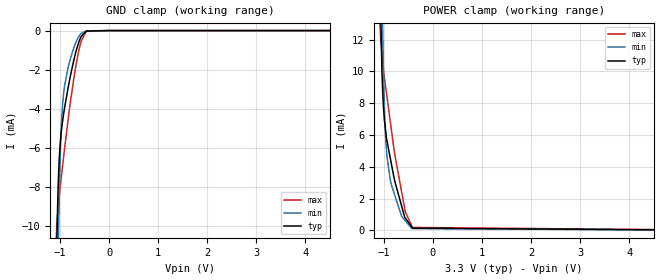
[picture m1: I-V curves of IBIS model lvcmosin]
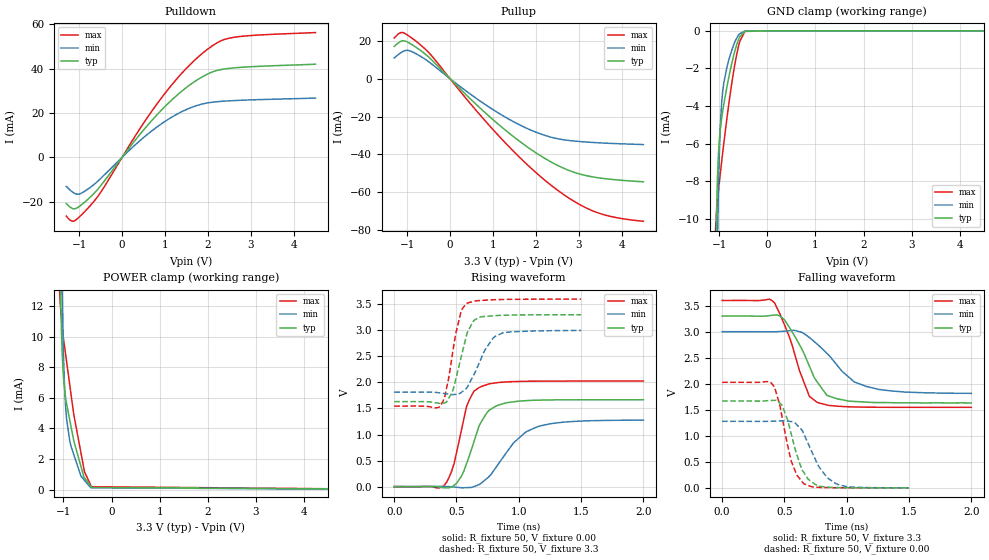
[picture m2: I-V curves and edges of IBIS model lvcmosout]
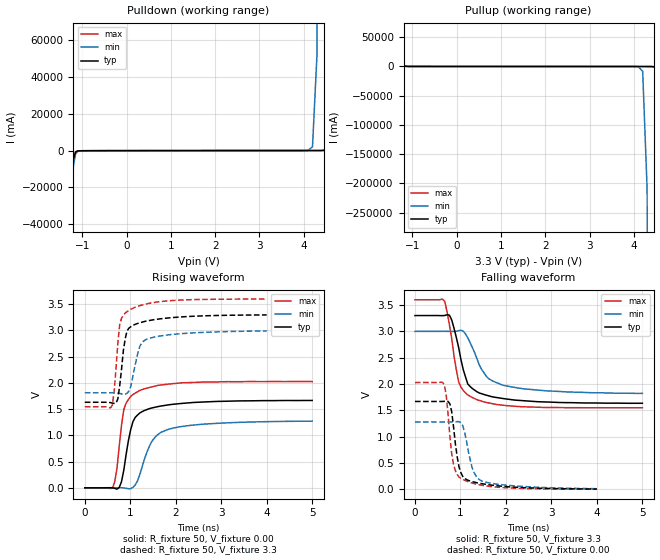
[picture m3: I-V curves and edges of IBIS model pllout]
|Texas Instruments, Incorporated   |
|Four Output Clock Generator/Jitter Cleaner With Integrated Dual VCOs   |
| Marketing part#   Voltage Range   Package-type   #pins/pkg drawing |
| CDCE62002RHBR   3.0V - 3.6V   QFN   32-pin RHB   |
| CDCE62002RHBT   3.0V - 3.6V   QFN   32-pin RHB   |
[IBIS Ver]   4.0
[File name]   cdce62002.ibs
[File Rev]   1.0
[Date]   09/18/2015
[Source]   Texas Instruments Incorporated.
   Analog-eLab, HPA
   12500 TI Blvd
   Dallas, TX -75243
   For Support e-mail: elab_scm_ibis@list.ti.com
[Notes]   Revision History
   Rev 1.0: 09/18/2015
   - Same base die and models as CDCE62005, new package model.
[Disclaimer] This model is designed as an aid for customers of Texas Instruments.
 TI and its licensors and suppliers make no warranties, either expressed
 or implied, with respect to this  model, including the warranties of
 merchantability or fitness for a particular purpose.
 The model is provided solely on an "as is" basis. The entire risk as to
 its quality and performance is with the customer.
[Copyright] (C)Copyright 2015 Texas Instruments Incorporated.
   All rights reserved.
|   Component   CDCE62002RHB
[Component]   CDCE62002RHB
[Manufacturer]   Texas Instruments Incorporated
[Package]   |32-pin RHB Package, QFN
|   typ   min   max
R_pkg   0.1266   0.0917   0.1676
L_pkg   1.089nH   0.7569nH   1.4898nH
C_pkg   0.1201pF   0.0925pF   0.1533pF
[Pin] signal_name   model_name   R_pin   L_pin   C_pin
1   VCC_AUX   POWER   0.00505   0.15571nH   1.25602pF
2   AUX_IN   lvcmosin   0.13153   1.1302nH   0.1258pF
3   VBB   POWER   0.10832   0.90731nH   0.10655pF
4   VCC_PLLD   POWER   0.04958   0.55167nH   0.12597pF
5   REG_CAP1   NC   0.09166   0.75685nH   0.09254pF
6   PDN   lvcmosin   0.09642   0.80223nH   0.09606pF
7   SPI_MISO   lvcmosout   0.11258   0.95481nH   0.10947pF
8   SPI_MOSI   lvcmosin   0.13603   1.18504nH   0.11758pF
9   VCC_OUT0   POWER   0.07038   0.91081nH   0.16021pF
10   U0_N   univoutN   0.13453   1.1681nH   0.12847pF
11   U0_P   univoutP   0.13111   1.13436nH   0.12596pF
12   VCC_OUT1   POWER   0.06752   0.84332nH   0.17642pF
13   VCC_OUT2   POWER   0.06751   0.84583nH   0.17926pF
14   U1_N   univoutN   0.13123   1.13557nH   0.12556pF
15   U1_P   univoutP   0.13419   1.1648nH   0.12877pF
16   VCC_OUT3   POWER   0.0704   0.90108nH   0.16069pF
17   SPI_CLK   lvcmosin   0.13766   1.20093nH   0.1195pF
18   SPI_LE   lvcmosin   0.11212   0.95041nH   0.11038pF
19   TEST_SYNC   NC   0.09475   0.78685nH   0.09573pF
20   REG_CAP3   NC   0.09303   0.76838nH   0.09454pF
21   GND_PLLDIV   GND   0.05226   0.59794nH   0.13463pF
22   VCC_PLLDIV   POWER   0.05772   0.69812nH   0.14663pF
23   REG_CAP4   NC   0.13319   1.1464nH   0.12871pF
24   VCC_VCO   POWER   0.07578   1.10044nH   0.15548pF
25   EXT_LF_P   NC   0.16761   1.48983nH   0.15332pF
26   EXT_LF_N   NC   0.14699   1.2821nH   0.13427pF
27   REG_CAP2   NC   0.13767   1.18956nH   0.13285pF
28   VCC_PLLA   POWER   0.06718   0.82907nH   0.17636pF
29   REF_P   univin   0.13272   1.14077nH   0.12791pF
30   REF_N   univin   0.13255   1.13927nH   0.12699pF
31   VCC_IN   POWER   0.06896   0.86472nH   0.17429pF
32   PLL_LOCK   pllout   0.14347   1.24974nH   0.12652pF
|33   GND_THERMALPAD
[Diff Pin]  inv_pin  vdiff  tdelay_typ tdelay_min tdelay_max
| VDIFF TYP FOR lvds = 410mV; lvpecl_lo = 690mV
|lvpecl_hi = 810mV
11   10   0   NA   NA   NA
15   14   0   NA   NA   NA
29   30   200mV   NA   NA   NA
[Model Selector]   univoutP
univoutc   buffer with LVCMOS
univoutl   buffer with LVDS with normal swing
LVPECL_RC_HI_p LVPECL for HI SWING for positive Pin
LVPECL_RC_LO_p LVPECL for LO SWING for positive pin
[Model Selector]   univoutN
univoutc   buffer with LVCMOS
univoutl   buffer with LVDS with normal swing
LVPECL_RC_HI_n LVPECL for HI SWING for negative Pin
LVPECL_RC_LO_n LVPECL for LO SWING for negative pin
[Model Selector]   univin
univinc   input buffer with LVCMOS with internal termination
univine   input buffer with LVPECL with internal termination
univinl   input buffer with LVDS with internal termination
| Models and submodels in the file (12): lvcmosin (Input), lvcmosout (3-state), pllout (Output), univinc (Input), univinl (Input), univine (Input), univoutc (Output), LVPECL_RC_HI_p (Output_ECL), LVPECL_RC_HI_n (Output_ECL), LVPECL_RC_LO_p (Output_ECL), LVPECL_RC_LO_n (Output_ECL), univoutl (3-state)
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|   Model   lvcmosin
[Model]   lvcmosin
Model_type   Input
Polarity   Non-Inverting
Vinl   =   0.99V
Vinh   =   2.31V
|Variable   typ   min   max
C_comp   6.462e-13   6.387e-13   6.627e-13
[Model Spec]
Vinl   0.99V   0.9V   1.08V
Vinh   2.31V   2.1V   2.52V
|Variable   typ   min   max
[Voltage range]   3.3   3.0   3.6
|Variable   typ   min   max
[Temperature range]  25   85   0
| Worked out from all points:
|   GND clamp passes 1 mA (typ) near -0.67 V on its own axis
|   POWER clamp passes 1 mA (typ) near -0.59 V on its own axis
[GND Clamp]
|   Voltage   I(typ)   I(min)   I(max)
-3.3V     -1.163A    -1.155A    -1.183A
-1.077V   -12.52mA   -19.9mA    -10.51mA
-1.062V   -10.33mA   -16.3mA    -9.851mA
-1.04V    -8.005mA   -11.81mA   -9.112mA
-1.03V    -7.282mA   -10.19mA   -8.835mA
-1.001V   -5.883mA   -6.686mA   -8.1mA
-975.8mV  -5.179mA   -4.92mA    -7.525mA
-948.5mV  -4.618mA   -3.762mA   -6.913mA
-906.5mV  -3.923mA   -2.782mA   -5.998mA
-666.2mV  -976.2uA   -532.3uA   -1.635mA
-473.3mV  -43.09uA   -22.62uA   -64.41uA
6.598V    0A         0A         0A
[POWER Clamp]
|   Voltage   I(typ)   I(min)   I(max)
-3.3V     1.174A     1.165A     1.197A
-1.079V   16.53mA    24.99mA    12.95mA
-1.065V   13.88mA    21.26mA    12.05mA
-1.025V   8.881mA    12.83mA    10.64mA
-1.005V   7.625mA    9.46mA     9.995mA
-990.5mV  6.997mA    7.918mA    9.669mA
-956.5mV  6.058mA    5.501mA    8.88mA
-866.6mV  4.514mA    3.149mA    6.797mA
-778.6mV  3.136mA    2.225mA    4.803mA
-562.5mV  777.7uA    608.5uA    1.165mA
-432.4mV  233.3uA    121.2uA    290.1uA
6.59V     0A         0A         0A
|   Model   lvcmosout
[Model]   lvcmosout
Model_type   3-state
Polarity   Non-Inverting
Enable   Active-Low
Vmeas  =   1.55V
Cref   =   5pF
Vref   =   0V
|Variable   typ   min   max
C_comp   1.519e-12   1.481e-12   1.560e-12
[Model Spec]
Vmeas   1.55V   1.4V   1.7V
|Variable   typ   min   max
[Voltage range]   3.3   3.0   3.6
|Variable   typ   min   max
[Temperature range]  25   85   0
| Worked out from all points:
|   slope of the pulldown table from 0 to 0.495 V, typ, clamps not added: 40.6 ohm
|   slope of the pullup table from 0 to 0.495 V, typ, clamps not added: 44.4 ohm
|   GND clamp passes 1 mA (typ) near -0.67 V on its own axis
|   POWER clamp passes 1 mA (typ) near -0.59 V on its own axis
|   rising waveform, R_fixture 50, V_fixture 0.00: 20-80 % time 158ps typ, 259ps min, 120ps max; typ from 0 V to 1.67 V
|   falling waveform, R_fixture 50, V_fixture 3.3: 20-80 % time 215ps typ, 291ps min, 178ps max; typ from 3.3 V to 1.63 V
|   rising waveform, R_fixture 50, V_fixture 3.3: 20-80 % time 104ps typ, 150ps min, 92.8ps max; typ from 1.63 V to 3.3 V
|   falling waveform, R_fixture 50, V_fixture 0.00: 20-80 % time 125ps typ, 166ps min, 114ps max; typ from 1.67 V to 0 V
[Pulldown]
|Voltage   I(typ)   I(min)   I(max)
-1.3V     -20.86mA   -13.1mA    -26.48mA
-1.1V     -23.23mA   -16.33mA   -28.55mA
-950mV    -21.45mA   -16.2mA    -26.02mA
-700mV    -17.18mA   -12.95mA   -20.87mA
-450mV    -11.61mA   -8.626mA   -14.35mA
300mV     7.577mA    5.517mA    9.454mA
900mV     20.95mA    14.87mA    26.35mA
1.45V     30.75mA    21.11mA    39.14mA
2V        37.61mA    24.53mA    48.85mA
2.3V      39.52mA    25.19mA    52.48mA
2.6V      40.28mA    25.55mA    54.06mA
4.5V      41.95mA    26.7mA     56.2mA
[Pullup]
|Voltage   I(typ)   I(min)   I(max)
-1.3V     17.09mA    10.97mA    21.5mA
-1.2V     19.05mA    12.87mA    23.8mA
-1.1V     20.09mA    14.4mA     24.42mA
-950mV    18.9mA     14.88mA    22.47mA
-600mV    13.46mA    10.63mA    16.14mA
450mV     -10.16mA   -7.788mA   -12.55mA
1.2V      -25.55mA   -19.16mA   -31.85mA
1.9V      -37.71mA   -27.37mA   -47.63mA
2.5V      -45.82mA   -31.73mA   -58.95mA
2.9V      -49.62mA   -33mA      -65.06mA
3.4V      -52.25mA   -33.84mA   -70.62mA
4.5V      -54.53mA   -34.84mA   -75.45mA
[GND Clamp]
|   Voltage   I(typ)   I(min)   I(max)
-3.3V     -1.163A    -1.155A    -1.183A
-1.077V   -12.52mA   -19.9mA    -10.51mA
-1.062V   -10.33mA   -16.3mA    -9.851mA
-1.04V    -8.005mA   -11.81mA   -9.112mA
-1.03V    -7.282mA   -10.19mA   -8.835mA
-1.001V   -5.883mA   -6.686mA   -8.1mA
-975.8mV  -5.179mA   -4.92mA    -7.525mA
-948.5mV  -4.618mA   -3.762mA   -6.913mA
-906.5mV  -3.923mA   -2.782mA   -5.998mA
-666.2mV  -976.2uA   -532.3uA   -1.635mA
-473.3mV  -43.09uA   -22.62uA   -64.41uA
6.598V    0A         0A         0A
[POWER Clamp]
|   Voltage   I(typ)   I(min)   I(max)
-3.3V     1.174A     1.165A     1.197A
-1.079V   16.53mA    24.99mA    12.95mA
-1.065V   13.88mA    21.26mA    12.05mA
-1.025V   8.881mA    12.83mA    10.64mA
-1.005V   7.625mA    9.46mA     9.995mA
-990.5mV  6.997mA    7.918mA    9.669mA
-956.5mV  6.058mA    5.501mA    8.88mA
-866.6mV  4.514mA    3.149mA    6.797mA
-778.6mV  3.136mA    2.225mA    4.803mA
-562.5mV  777.7uA    608.5uA    1.165mA
-432.4mV  233.3uA    121.2uA    290.1uA
6.59V     0A         0A         0A
[Ramp]
|Variable   typ   min   max
dV/dt_r  1.0005/1.537e-10   0.7666/2.634e-10   1.2168/1.176e-10
dV/dt_f  1.0009/2.073e-10   0.7118/2.984e-10   1.2319/1.700e-10
R_load  =  50
[Rising Waveform]
R_fixture   =   50
V_fixture   =   0.00
V_fixture_min   =   0.00
V_fixture_max   =   0.00
C_fixture   =   0.00
|Time   V(typ)   V(min)   V(max)
0s        0V         0V         0V
400ps     -23.73mV   2.624mV    20.83mV
480ps     23.97mV    -6.858mV   436.5mV
580ps     436.4mV    -19.51mV   1.532V
640ps     861.7mV    655.2uV    1.832V
700ps     1.248V     68.81mV    1.923V
820ps     1.55V      379.6mV    1.993V
960ps     1.629V     844.2mV    2.016V
1.16ns    1.659V     1.159V     2.025V
2ns       1.667V     1.276V     2.027V
[Falling Waveform]
R_fixture   =   50
V_fixture   =   3.3
V_fixture_min   =   3.0
V_fixture_max   =   3.6
C_fixture   =   0.00
|Time   V(typ)   V(min)   V(max)
0s        3.3V       3V         3.6V
420ps     3.319V     2.998V     3.558V
500ps     3.23V      3.01V      3.135V
580ps     2.925V     3.027V     2.592V
700ps     2.341V     2.889V     1.761V
760ps     2.046V     2.767V     1.647V
840ps     1.78V      2.587V     1.593V
1.06ns    1.66V      2.037V     1.554V
1.16ns    1.647V     1.947V     1.55V
2ns       1.631V     1.815V     1.547V
[Rising Waveform]
R_fixture   =   50
V_fixture   =   3.3
V_fixture_min   =   3.0
V_fixture_max   =   3.6
C_fixture   =   0.00
|Time   V(typ)   V(min)   V(max)
0s        1.631V     1.813V     1.546V
360ps     1.6V       1.801V     1.524V
405ps     1.606V     1.786V     1.716V
465ps     1.808V     1.766V     2.505V
540ps     2.511V     1.811V     3.392V
585ps     2.947V     1.901V     3.522V
645ps     3.2V       2.175V     3.561V
720ps     3.265V     2.585V     3.577V
810ps     3.282V     2.882V     3.588V
1.5ns     3.299V     2.998V     3.599V
[Falling Waveform]
R_fixture   =   50
V_fixture   =   0.00
V_fixture_min   =   0.00
V_fixture_max   =   0.00
C_fixture   =   0.00
|Time   V(typ)   V(min)   V(max)
0s        1.668V     1.278V     2.028V
375ps     1.677V     1.278V     2.042V
420ps     1.681V     1.282V     1.94V
480ps     1.59V      1.289V     1.376V
555ps     1.033V     1.273V     513.2mV
600ps     637.5mV    1.212V     245.4mV
660ps     279.2mV    1.014V     73.18mV
780ps     31.5mV     394.6mV    9.77mV
915ps     6.045mV    79.09mV    2.109mV
1.5ns     389.2uV    817.9uV    264.9uV
|   Model   pllout
[Model]   pllout
Model_type   Output
Polarity   Non-Inverting
Vmeas  =   1.55V
Cref   =   5pF
Vref   =   0V
|Variable   typ   min   max
C_comp   1.402e-12   1.338e-12   1.517e-12
[Model Spec]
Vmeas   1.55V   1.4V   1.7V
|Variable   typ   min   max
[Voltage range]   3.3   3.0   3.6
|Variable   typ   min   max
[Temperature range]  25   85   0
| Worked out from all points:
|   slope of the pulldown table from 0 to 0.495 V, typ, clamps not added: 40.6 ohm
|   slope of the pullup table from 0 to 0.495 V, typ, clamps not added: 44.5 ohm
|   rising waveform, R_fixture 50, V_fixture 0.00: 20-80 % time 246ps typ, 401ps min, 202ps max; typ from 0 V to 1.67 V
|   falling waveform, R_fixture 50, V_fixture 3.3: 20-80 % time 312ps typ, 488ps min, 259ps max; typ from 3.3 V to 1.63 V
|   rising waveform, R_fixture 50, V_fixture 3.3: 20-80 % time 152ps typ, 209ps min, 136ps max; typ from 1.63 V to 3.3 V
|   falling waveform, R_fixture 50, V_fixture 0.00: 20-80 % time 174ps typ, 228ps min, 165ps max; typ from 1.67 V to 0.003 V
[Pulldown]
|Voltage   I(typ)   I(min)   I(max)
-1.25V    -33.05A    -41.39A    -31.2A
-1.2V     -4.782A    -8.231A    -3.811A
-1.15V    -739.8mA   -1.667A    -530.3mA
-1.1V     -157.4mA   -364.2mA   -132mA
4.1V      48.21mA    119.9mA    56.69mA
4.2V      51.55mA    2.061A     59.35mA
4.3V      55.87mA    51.49A     62.81mA
4.4V      84.37mA    1.314kA    66.83mA
4.45V     229.9mA    6.639kA    69.02mA
[Pullup]
|Voltage   I(typ)   I(min)   I(max)
-1.3V     56.91A     51.48A     64.16A
-1.25V    8.169A     10.21A     7.723A
-1.2V     1.205A     2.048A     974.3mA
-1.15V    207.8mA    429.9mA    164mA
4.1V      -66.29mA   -382.4mA   -75.43mA
4.2V      -73.78mA   -8.251A    -79.41mA
4.3V      -84.22mA   -208.9A    -85.91mA
4.4V      -188.5mA   -5.334kA   -94.1mA
4.45V     -771.1mA   -26.96kA   -98.69mA
[Ramp]
|Variable   typ   min   max
dV/dt_r  1.0004/2.392e-10   0.7665/4.040e-10   1.2163/1.981e-10
dV/dt_f  1.0010/3.133e-10   0.7121/5.006e-10   1.2320/2.538e-10
R_load  =  50
[Rising Waveform]
R_fixture   =   50
V_fixture   =   0.00
V_fixture_min   =   0.00
V_fixture_max   =   0.00
C_fixture   =   0.00
|Time   V(typ)   V(min)   V(max)
0s        0V         0V         0V
606.1ps   1.735mV    3.233uV    -11.34mV
707.1ps   -25.63mV   1.211mV    369mV
808.1ps   119mV      1.517mV    1.194V
858.6ps   338.8mV    -1.533mV   1.496V
1.01ns    1.112V     -17.3mV    1.744V
1.212ns   1.428V     257.6mV    1.857V
1.465ns   1.52V      871.2mV    1.923V
1.869ns   1.585V     1.123V     1.98V
5ns       1.666V     1.271V     2.027V
[Falling Waveform]
R_fixture   =   50
V_fixture   =   3.3
V_fixture_min   =   3.0
V_fixture_max   =   3.6
C_fixture   =   0.00
|Time   V(typ)   V(min)   V(max)
0s        3.3V       3V         3.599V
656.6ps   3.301V     3V         3.564V
808.1ps   3.216V     2.998V     2.864V
959.6ps   2.696V     3.012V     2.043V
1.061ns   2.276V     3.005V     1.878V
1.162ns   1.998V     2.877V     1.791V
1.263ns   1.912V     2.691V     1.741V
1.566ns   1.788V     2.151V     1.649V
1.97ns    1.719V     1.969V     1.593V
5ns       1.633V     1.821V     1.546V
[Rising Waveform]
R_fixture   =   50
V_fixture   =   3.3
V_fixture_min   =   3.0
V_fixture_max   =   3.6
C_fixture   =   0.00
|Time   V(typ)   V(min)   V(max)
0s        1.631V     1.812V     1.546V
606.1ps   1.615V     1.813V     1.576V
646.5ps   1.61V      1.813V     1.844V
727.3ps   1.696V     1.807V     2.763V
767.7ps   1.946V     1.8V       3.109V
888.9ps   2.843V     1.788V     3.333V
969.7ps   3.043V     1.842V     3.382V
1.212ns   3.148V     2.701V     3.474V
1.333ns   3.176V     2.822V     3.501V
4ns       3.296V     2.991V     3.599V
[Falling Waveform]
R_fixture   =   50
V_fixture   =   0.00
V_fixture_min   =   0.00
V_fixture_max   =   0.00
C_fixture   =   0.00
|Time   V(typ)   V(min)   V(max)
0s        1.667V     1.278V     2.027V
646.5ps   1.67V      1.277V     1.986V
686.9ps   1.676V     1.277V     1.787V
767.7ps   1.622V     1.278V     1.001V
848.5ps   1.182V     1.281V     469.1mV
929.3ps   611.1mV    1.284V     278.7mV
1.01ns    313.4mV    1.259V     206.8mV
1.293ns   137.2mV    326.8mV    109.4mV
1.495ns   101.5mV    144.3mV    71.88mV
4ns       3.49mV     9.898mV    878.2uV
